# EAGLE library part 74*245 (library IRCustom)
Octal BUS TRANSCEIVER, 3-state
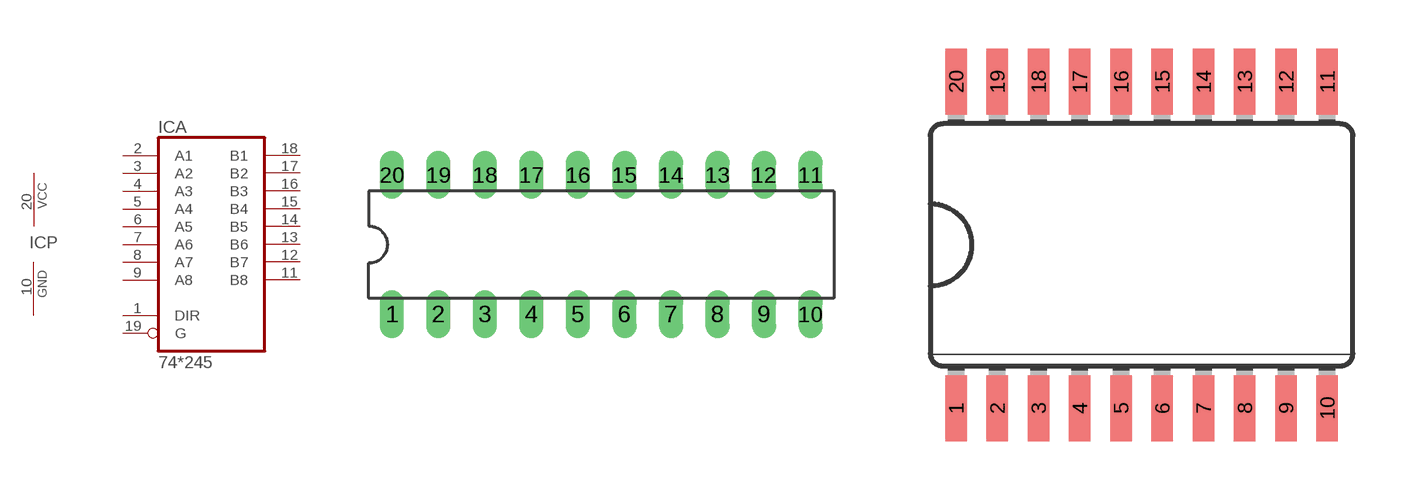
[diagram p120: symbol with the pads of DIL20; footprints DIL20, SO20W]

Designator prefix IC; gates A=74245 P=PWRN

## 74LS245N  [DIL20]
1  A:DIR  in
2  A:A1
3  A:A2
4  A:A3
5  A:A4
6  A:A5
7  A:A6
8  A:A7
9  A:A8
10  P:GND  pwr
11  A:B8
12  A:B7
13  A:B6
14  A:B5
15  A:B4
16  A:B3
17  A:B2
18  A:B1
19  A:G  in
20  P:VCC  pwr

## 74LS245DW  [SO20W]
Pads as for DIL20

## 74LS245FK  [LCC20]
Pads as for DIL20

## 74245MTC  [SSOP20]
Pads as for DIL20

## Footprint DIL20 (pad centres in mm)
Dual In Line Package
drill 0.813 long: 1 -11.43,-3.81; 2 -8.89,-3.81; 3 -6.35,-3.81; 4 -3.81,-3.81; 5 -1.27,-3.81; 6 1.27,-3.81; 7 3.81,-3.81; 8 6.35,-3.81; 9 8.89,-3.81; 10 11.43,-3.81; 11 11.43,3.81; 12 8.89,3.81; 13 6.35,3.81; 14 3.81,3.81; 15 1.27,3.81; 16 -1.27,3.81; 17 -3.81,3.81; 18 -6.35,3.81; 19 -8.89,3.81; 20 -11.43,3.81

## Footprint SO20W (pad centres in mm)
Wide Small Outline package 300 mil
smd 0.66 x 2.032: 1 -5.715,-5.029; 2 -4.445,-5.029; 3 -3.175,-5.029; 4 -1.905,-5.029; 5 -0.635,-5.029; 6 0.635,-5.029; 7 1.905,-5.029; 8 3.175,-5.029; 9 4.445,-5.029; 10 5.715,-5.029; 11 5.715,5.029; 12 4.445,5.029; 13 3.175,5.029; 14 1.905,5.029; 15 0.635,5.029; 16 -0.635,5.029; 17 -1.905,5.029; 18 -3.175,5.029; 19 -4.445,5.029; 20 -5.715,5.029

## Footprint LCC20 (pad centres in mm)
Leadless Chip Carrier Ceramic Package
smd 0.8 x 3.4: 1 0,3.8
smd 0.8 x 2: 2 -1.27,4.5; 3 -2.54,4.5; 9 -2.54,-4.5; 10 -1.27,-4.5; 11 0,-4.5; 12 1.27,-4.5; 13 2.54,-4.5; 19 2.54,4.5; 20 1.27,4.5
smd 2 x 0.8: 4 -4.5,2.54; 5 -4.5,1.27; 6 -4.5,0; 7 -4.5,-1.27; 8 -4.5,-2.54; 14 4.5,-2.54; 15 4.5,-1.27; 16 4.5,0; 17 4.5,1.27; 18 4.5,2.54

## Footprint SSOP20 (pad centres in mm)
smd 0.4 x 1.8: 1 -2.925,-3; 2 -2.275,-3; 3 -1.625,-3; 4 -0.975,-3; 5 -0.325,-3; 6 0.325,-3; 7 0.975,-3; 8 1.625,-3; 9 2.275,-3; 10 2.925,-3; 11 2.925,3; 12 2.275,3; 13 1.625,3; 14 0.975,3; 15 0.325,3; 16 -0.325,3; 17 -0.975,3; 18 -1.625,3; 19 -2.275,3; 20 -2.925,3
